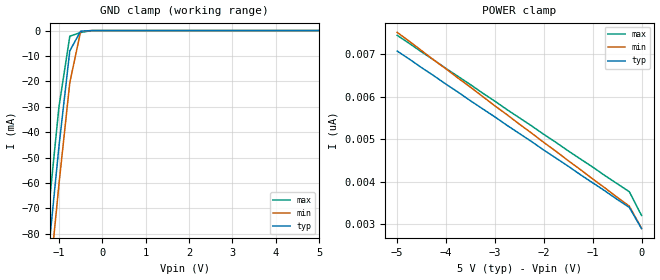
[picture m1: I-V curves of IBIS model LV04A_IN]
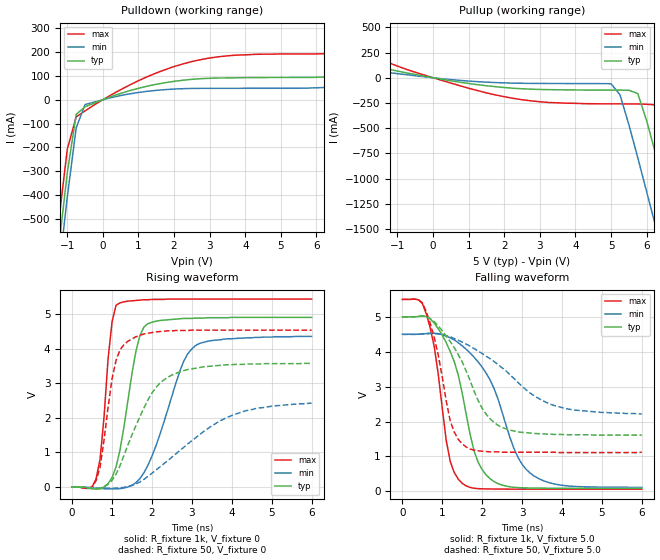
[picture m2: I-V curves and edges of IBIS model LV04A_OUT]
| Copyright 2000, Texas Instruments Inc., All Rights Reserved.
|<HTML><HEAD><TITLE>TI SN74LV04A IBIS Model</TITLE></HEAD><BODY><H1>
| Texas Instruments Incorporated</H1><B>
| Standard Linear and Logic Group<BR>
| IBIS Model of SN74LV04A<BR>
| HEX INVERTER<BR>
| SOIC 14-pin (D) Package<BR></B><HR><PRE>
[IBIS Ver]   2.1
[Comment Char]  <_char
[File Name]   lv04html.ibs
[File Rev]   2.0
[Date]   February 29, 2000
[Source]   Data created from HSPICE simulations at TI-SLL.
[Notes]   For questions and comments concerning SLL IBIS models, please
   email: <a href="mailto:sllibis@ti.com">sllibis@ti.com</a>
<HR>
[Disclaimer] </PRE><BLOCKQUOTE>
<P>Property of Texas Instruments Incorporated.  Unauthorized reproduction
 and/or distribution is strictly prohibited.</P>
<P>This product is protected under copyright law. Created 2000, &copy;
 Copyright 2000, Texas Instruments Inc., All Rights Reserved.</P>
<P><B>UNLESS THERE IS A SIGNED, WRITTEN AGREEMENT TO THE CONTRARY,
TEXAS INSTRUMENTS (TI) IS PROVIDING THE IBIS MODELS  AND WITHOUT ANY
WARRANTY, EXPRESSED OR IMPLIED.</B></P>
<P>TI assumes no liability for:</P><OL>
<LI>the accuracy of the IBIS models provided to your company;</LI>
<LI>the proper functioning of these IBIS Models in your design or for
any resulting applications; or</LI>
<LI>infringement of patents, copyrights or intellectual property rights
 resulting from your use of these IBIS models.</LI></OL>
<P>TI provides IBIS Models as a service to our customers. You and your
 company shall not distribute, sell or give these models to anyone else
 without prior written permission from TI.</P>
<P>TI reserves the right to make changes to our products or to discontinue
 any semiconductor product or service without notice, and advises our
 customers to obtain the latest version of relevant information to verify,
 before placing orders, that the information being relied on is current.</P>
<P>Please be aware that your receipt and use of the IBIS information
 provided shall serve as acceptance of these terms and conditions. If you
 do not accept these terms, you should return or destroy the IBIS models
 and any other accompanying information immediately.<P></BLOCKQUOTE>
</PRE><HR><H3><CENTER>LV04A Component</CENTER></H3><PRE>
[Component]   LV04A
[Manufacturer]   Texas Instruments, Inc.
[Package]
<BR>   typ   min   max
R_pkg   0.031   0.028   0.034
L_pkg   3.109nH   2.462nH   3.889nH
C_pkg   0.473pF   0.363pF   0.628pF
<BR>
<IMG SRC="pinout.gif">
[Pin]   signal_name   model_name   R_pin   L_pin   C_pin
<BR>
1   1A   LV04A_IN   0.033   3.854nH   0.622pF
2   1Y   LV04A_OUT   0.032   3.188nH   0.473pF
3   2A   LV04A_IN   0.028   2.462nH   0.377pF
4   2Y   LV04A_OUT   0.031   2.596nH   0.363pF
5   3A   LV04A_IN   0.028   2.521nH   0.372pF
6   3Y   LV04A_OUT   0.034   3.250nH   0.476pF
7   GND   GND   0.034   3.889nH   0.628pF
8   4Y   LV04A_OUT   0.034   3.889nH   0.628pF
9   4A   LV04A_IN   0.034   3.250nH   0.476pF
10   5Y   LV04A_OUT   0.028   2.521nH   0.372pF
11   5A   LV04A_IN   0.031   2.596nH   0.364pF
12   6Y   LV04A_OUT   0.028   2.462nH   0.377pF
13   6A   LV04A_IN   0.032   3.188nH   0.473pF
14   VCC   POWER   0.033   3.854nH   0.622pF
< Models and submodels in the file (2): LV04A_IN (Input), LV04A_OUT (Output)
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<table border><tr><td colspan="2"><b><center>Function Table</center></b></tr>
<tr><td><b>Input A</b></td><td><b>Output Y</b></td></tr>
<tr><td>H</td><td>L</td></tr>
<tr><td>L</td><td>H</td></tr></table>
<IMG SRC="logic.gif">
</PRE><HR><H3><CENTER>LV04A_IN Model</CENTER></H3><PRE>
[Model]   LV04A_IN
Model_type  Input
Polarity   Non-Inverting
Vinl = 1.5
Vinh = 3.5
<BR>
<BR>variable   typ   min   max
C_comp   1.23pf   0.93pf   1.53pf
<BR>
[Temperature Range]   25   85   -40
[Voltage range]   5.0   4.5   5.5
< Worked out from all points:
<   GND clamp passes 1 mA (typ) near -0.52 V on its own axis
<BR>
[GND Clamp]
<BR>
<BR>   Voltage   I(typ)   I(min)   I(max)
<BR>
-5V       -773mA     -786mA     -758mA
-1.5V     -133mA     -148mA     -117mA
-1.25V    -88.7mA    -104mA     -72.7mA
-1V       -45.6mA    -60.5mA    -30mA
-750mV    -7.99mA    -20.5mA    -2.23mA
-500mV    -233uA     -353uA     -759uA
-250mV    -2.63nA    -182nA     -26.9uA
5V        2.9nA      3.64nA     2.54nA
<BR>
[POWER Clamp]
<BR>
<BR>   Voltage   I(typ)   I(min)   I(max)
<BR>
-5V       7.08nA     7.52nA     7.45nA
-1.5V     4.37nA     4.5nA      4.73nA
-250mV    3.4nA      3.43nA     3.77nA
0V        2.9nA      2.91nA     3.21nA
</PRE><HR><H3><CENTER>LV04A_OUT Model</CENTER></H3><PRE>
[Model]   LV04A_OUT
Model_type  Output
Polarity   Inverting
Vmeas = 2.50v
Cref = 15pf
<IMG SRC="pmi.gif">
<BR>variable   typ   min   max
C_comp   4.62pf   3.47pf   5.77pf
<BR>
[Temperature Range]   25   85   -40
[Voltage range]   5.0   4.5   5.5
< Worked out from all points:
<   slope of the pulldown table from 0 to 0.75 V, typ, clamps not added: 19.8 ohm
<   slope of the pullup table from 0 to 0.75 V, typ, clamps not added: 17.2 ohm
<   rising waveform, R_fixture 1k, V_fixture 0: 20-80 % time 416ps typ, 751ps min, 237ps max; typ from 0 V to 4.91 V
<   rising waveform, R_fixture 50, V_fixture 0: 20-80 % time 858ps typ, 1.66ns min, 352ps max; typ from 0 V to 3.58 V
<   falling waveform, R_fixture 1k, V_fixture 5.0: 20-80 % time 629ps typ, 934ps min, 401ps max; typ from 5 V to 0.085 V
<   falling waveform, R_fixture 50, V_fixture 5.0: 20-80 % time 874ps typ, 1.53ns min, 461ps max; typ from 5 V to 1.61 V
<BR>
[Pulldown]
<BR>
<BR>   Voltage   I(typ)   I(min)   I(max)
<BR>
-5V       -5.86A     -5.96A     -5.76A
-1.5V     -969mA     -1.07A     -859mA
-1.25V    -631mA     -736mA     -522mA
-1V       -307mA     -409mA     -208mA
-750mV    -61.5mA    -118mA     -72.1mA
-500mV    -29.4mA    -20.1mA    -46.7mA
1V        48mA       30.4mA     79.8mA
2.5V      85.4mA     47.3mA     160mA
3.75V     91.9mA     47.8mA     187mA
6V        94mA       49.9mA     192mA
7V        104mA      57.2mA     202mA
10V       164mA      87.8mA     302mA
<BR>
[Pullup]
<BR>
<BR>   Voltage   I(typ)   I(min)   I(max)
<BR>
-5V       228mA      118mA      489mA
-3.25V    214mA      116mA      410mA
-500mV    32.9mA     20.4mA     54.7mA
1.75V     -88.5mA    -47.6mA    -170mA
5V        -123mA     -59mA      -259mA
5.25V     -123mA     -168mA     -259mA
5.75V     -156mA     -792mA     -260mA
6.25V     -752mA     -1.47A     -269mA
6.5V      -1.09A     -1.82A     -452mA
6.75V     -1.43A     -2.16A     -777mA
7.25V     -2.13A     -2.86A     -1.46A
10V       -5.98A     -6.72A     -5.32A
<BR>
[Ramp]
<BR>
<BR>variable   typ   min   max
dV/dt_r   2.97E+00/4.90E-10   2.64E+00/8.10E-10   3.28E+00/2.46E-10
dV/dt_f   2.97E+00/7.19E-10   2.65E+00/1.01E-09   3.28E+00/4.80E-10
R_load = 1k
<BR>
[Rising Waveform]
R_fixture = 1k
V_fixture = 0
<BR>
<BR>   Time   V(typ)   V(min)   V(max)
<BR>
0s        0V         0V         0V
600ps     -62.9mV    -38.3mV    233mV
700ps     -50.3mV    -44.7mV    800mV
1ns       273mV      -56.3mV    4.78V
1.1ns     579mV      -55mV      5.26V
1.6ns     3.94V      127mV      5.4V
1.9ns     4.73V      632mV      5.42V
2.8ns     4.88V      3.65V      5.44V
3.1ns     4.89V      4.1V       5.44V
6ns       4.91V      4.36V      5.44V
<BR>
[Rising Waveform]
R_fixture = 50
V_fixture = 0
<BR>
<BR>   Time   V(typ)   V(min)   V(max)
<BR>
0s        0V         0V         0V
600ps     -46.8mV    -27.9mV    184mV
700ps     -33.2mV    -30.8mV    571mV
1ns       194mV      -34.9mV    3.13V
1.1ns     369mV      -31.9mV    3.66V
1.4ns     1.22V      11.6mV     4.22V
2ns       2.72V      399mV      4.47V
2.5ns     3.24V      863mV      4.52V
4ns       3.54V      2.07V      4.54V
6ns       3.58V      2.43V      4.54V
<BR>
[Falling Waveform]
R_fixture = 1k
V_fixture = 5.0
V_fixture_min = 4.5
V_fixture_max = 5.5
<BR>
<BR>   Time   V(typ)   V(min)   V(max)
<BR>
0s        5V         4.5V       5.5V
600ps     5.01V      4.52V      5.09V
800ps     4.82V      4.53V      4.15V
1.2ns     4.01V      4.4V       858mV
1.5ns     2.82V      4.17V      229mV
1.8ns     1.15V      3.84V      86.6mV
2ns       622mV      3.56V      70.7mV
2.8ns     115mV      1.22V      61.9mV
3.2ns     94.7mV     525mV      61.3mV
6ns       84.9mV     113mV      61.5mV
<BR>
[Falling Waveform]
R_fixture = 50
V_fixture = 5.0
V_fixture_min = 4.5
V_fixture_max = 5.5
<BR>
<BR>   Time   V(typ)   V(min)   V(max)
<BR>
0s        5V         4.5V       5.5V
400ps     5.01V      4.5V       5.49V
600ps     5.01V      4.52V      5.15V
900ps     4.74V      4.51V      3.91V
1.2ns     4.29V      4.43V      2.02V
1.6ns     3.45V      4.22V      1.27V
2ns       2.38V      3.95V      1.15V
2.5ns     1.83V      3.54V      1.12V
3.8ns     1.63V      2.46V      1.12V
6ns       1.61V      2.22V      1.12V
